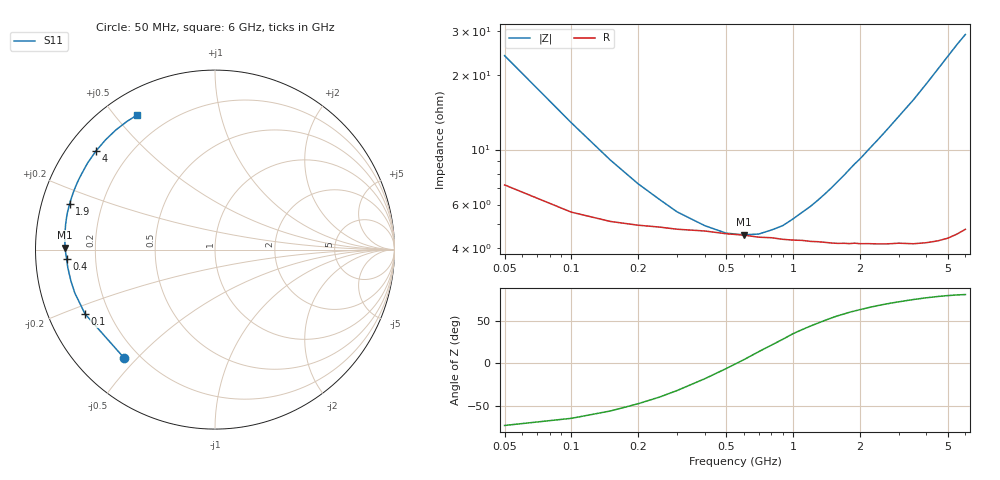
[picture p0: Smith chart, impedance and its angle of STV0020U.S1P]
! SIEMENS Discrete & RF Semiconductors
! BA892
! Si PIN Diode in SCD-80
! IF = 0.02 mA
! S-Parameters:  September  1997
# GHz  S  MA  R  50
!  f  S11
! GHz  MAG  ANG
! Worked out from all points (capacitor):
!   34 points, 50 MHz to 6 GHz, reference 50 ohm
!   read as one part to ground: C = 133 pF near 50 MHz
!   lowest |Z| = 4.53 ohm at 600 MHz (marker M1)
!   series resonance near 557.9 MHz, so ESL is about 610 pH
!   S11 on the Smith chart (normalised r, x): 50 MHz: 0.14, -0.46; 100 MHz: 0.11, -0.23; 400 MHz: 0.09, -0.03; 1.9 GHz: 0.08, +0.15; 4 GHz: 0.08, +0.36; 6 GHz: 0.10, +0.57
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0.05  0.7875 -130.2
0.1  0.8081 -153.7
0.15  0.8176 -162.8
0.2  0.8216 -167.7
0.25  0.8236 -170.8
0.3  0.8263 -173.2
0.4  0.8285 -176.5
0.5  0.8324 -178.9
0.6  0.8343 179.2
0.7  0.8372 177.5
0.8  0.8381 176.0
0.9  0.8404 174.6
1  0.8417 173.1
1.1  0.8423 171.8
1.2  0.8439 170.6
1.4  0.8457 168.2
1.6  0.8477 165.8
1.9  0.8486 162.4
2  0.8496 161.4
2.4  0.8518 157.1
2.8  0.8537 152.9
3  0.8544 150.8
3.5  0.8584 145.7
4  0.8612 140.3
4.5  0.8637 134.9
5  0.8657 129.6
5.5  0.8664 124.5
6  0.8664 119.9
